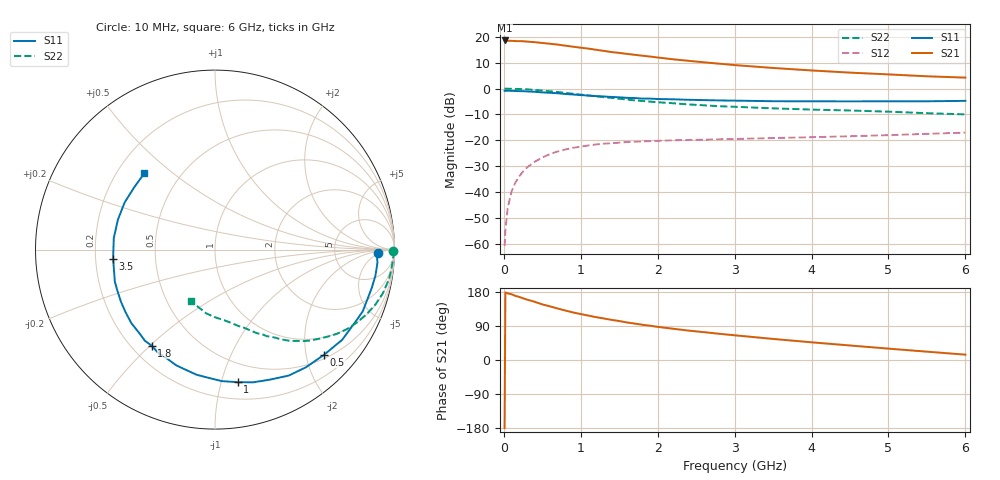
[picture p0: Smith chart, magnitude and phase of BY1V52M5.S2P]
! SIEMENS Small Signal Semiconductors
! BFY420
! Si NPN RF SIEGET Grounded Emitter Transistor in MICRO-X
! VCE = 1.5 V  IC = 2.5 mA
! Common Emitter S-Parameters:  October  1996
# GHz  S  MA  R  50
!  f  S11  S21  S12  S22
! GHz  MAG  ANG  MAG  ANG  MAG  ANG  MAG  ANG
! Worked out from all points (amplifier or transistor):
!   36 points, 10 MHz to 6 GHz, reference 50 ohm
!   highest |S21| = 18.6 dB at 10 MHz (marker M1)
!   |S21| within 3 dB of that: start of sweep to 1.058 GHz
!   unconditionally stable (mu >= 1): 3.78 GHz to end of sweep
!   at 250 MHz: K = 0.06, MSG = 25.2 dB, |S12| = -32.0 dB
!   at 1.4 GHz: K = 0.35, MSG = 17.6 dB, |S12| = -21.1 dB
!   at 6 GHz: K = 1.23, MAG = 7.7 dB, |S12| = -17.0 dB
!   S11 on the Smith chart (normalised r, x): 10 MHz: 20, -4; 500 MHz: 0.58, -2.36; 1 GHz: 0.34, -1.13; 1.8 GHz: 0.28, -0.51; 3.5 GHz: 0.27, -0.04; 6 GHz: 0.31, +0.40
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0.01  0.906 -1.1  8.521 -179.7  0.0009 103.2  0.9941 -0.5
0.02  0.9023 -2.1  8.511 178.3  0.0018 86.4  0.995 -0.9
0.05  0.9082 -4.6  8.365 176.0  0.0049 90.5  0.994 -2.4
0.1  0.9055 -9.3  8.377 173.5  0.0102 86.3  0.9903 -4.9
0.15  0.8991 -13.7  8.288 169.1  0.0153 81.1  0.9867 -7.4
0.2  0.8931 -18.2  8.275 166.5  0.0201 80.1  0.9829 -9.7
0.25  0.8921 -22.7  8.224 162.8  0.025 76.9  0.9737 -12.1
0.4  0.8686 -35.4  7.899 153.7  0.0385 69.7  0.9443 -19.0
0.5  0.8443 -43.9  7.615 146.7  0.0465 65.1  0.9169 -23.3
0.7  0.8133 -59.6  7.086 135.9  0.0608 57.1  0.858 -31.1
0.8  0.7866 -67.1  6.758 130.5  0.0666 52.9  0.8259 -34.6
1  0.7493 -80.3  6.175 121.2  0.0754 46.5  0.7645 -40.5
1.1  0.7338 -87.0  5.931 117.1  0.0797 43.9  0.7363 -43.4
1.4  0.6892 -103.7  5.082 105.9  0.0879 36.8  0.6617 -50.3
1.6  0.6624 -114.1  4.678 99.1  0.0926 33.1  0.6147 -54.1
1.8  0.6411 -123.4  4.32 93.0  0.095 30.1  0.5771 -57.4
2.2  0.6207 -138.7  3.684 82.5  0.1001 25.3  0.5212 -63.3
2.8  0.5902 -157.2  3.031 69.2  0.1048 21.2  0.4561 -70.7
3.5  0.57 -174.9  2.504 55.6  0.1107 18.2  0.4153 -78.1
4.5  0.5661 163.1  2.036 38.3  0.12 15.1  0.3772 -90.0
5.5  0.5684 142.4  1.729 22.0  0.1334 12.3  0.335 -105.5
6  0.5796 132.7  1.63 14.1  0.1411 10.7  0.3171 -114.7
